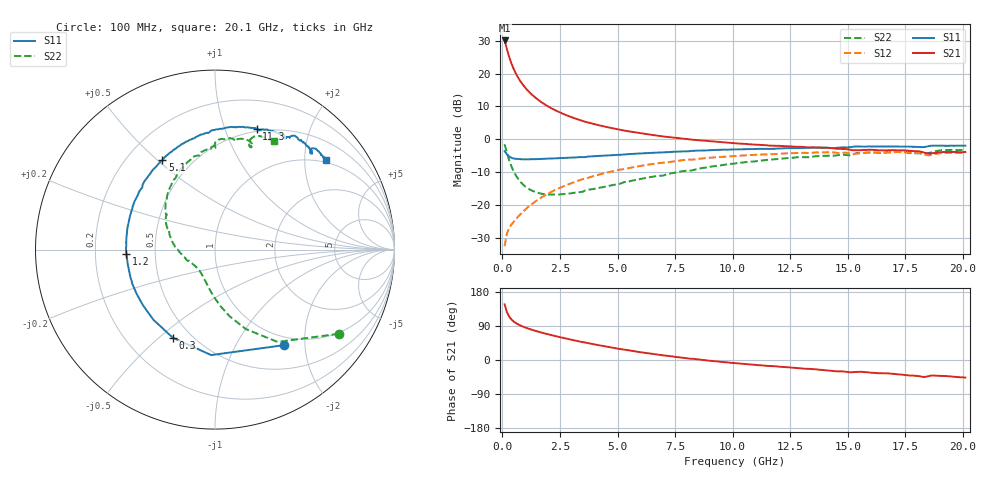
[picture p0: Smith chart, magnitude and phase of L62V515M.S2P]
!  Infineon Technologies AG
! BFR380L3 , PF131585-7, No.6, Th 09.10.01, soldered on pcb-board, measured with PP GSG850
!  Vce=2.5 V,  Ic=15.0 mA
! Common Emitter S-Parameters:  15. November 2001
#  GHz  S  MA  R  50
! f  S11  S21  S12  S22
! GHz  Mag  Ang  Mag  Ang  Mag  Ang  Mag  Ang
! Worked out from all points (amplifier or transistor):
!   201 points, 100 MHz to 20.1 GHz, reference 50 ohm
!   highest |S21| = 30.1 dB at 100 MHz (marker M1)
!   |S21| within 3 dB of that: start of sweep to 214.9 MHz
!   unconditionally stable (mu >= 1): 1.562 GHz to 4.486 GHz
!   at 3.4 GHz: K = 1.02, MAG = 8.2 dB, |S12| = -12.4 dB
!   at 10.1 GHz: K = 0.96, MSG = 1.9 dB, |S12| = -5.1 dB
!   at 20.1 GHz: K = 0.99, MSG = 0.1 dB, |S12| = -4.1 dB
!   S11 on the Smith chart (normalised r, x): 100 MHz: 0.86, -1.60; 300 MHz: 0.40, -0.55; 1.2 GHz: 0.34, -0.02; 5.1 GHz: 0.35, +0.52; 11.3 GHz: 0.47, +1.29; 20.1 GHz: 0.92, +2.52
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0.1  0.656 -54.3  31.89 147.0  0.02344 67.1  0.8341 -34.2
0.2  0.588 -92.1  23.53 126.3  0.03661 55.2  0.6213 -55.9
0.3  0.5441 -115.7  17.81 114.4  0.04449 52.4  0.4746 -68.8
0.4  0.5201 -131.3  14.09 106.8  0.05021 51.8  0.3806 -77.6
0.5  0.5073 -142.2  11.59 101.2  0.05556 52.9  0.3187 -84.2
0.6  0.5016 -150.3  9.81 97.1  0.06122 54.3  0.2758 -89.5
0.7  0.4987 -157.0  8.5 93.6  0.06685 55.5  0.2444 -94.1
0.8  0.4955 -162.0  7.497 90.6  0.07274 56.9  0.2212 -98.1
0.9  0.4929 -166.7  6.699 88.0  0.07869 57.8  0.2033 -101.7
1  0.4929 -170.4  6.063 85.7  0.08481 58.7  0.1897 -105.2
1.2  0.4937 -177.0  5.093 81.4  0.09731 59.9  0.1706 -111.3
1.6  0.4976 172.7  3.87 74.1  0.123 60.9  0.1507 -122.0
2.1  0.5049 162.5  2.996 66.1  0.1556 60.4  0.1435 -133.1
2.7  0.5179 152.2  2.38 57.5  0.1946 58.3  0.1463 -145.1
3.5  0.5327 140.1  1.888 47.0  0.2464 54.3  0.1589 -157.0
5.1  0.5773 120.5  1.392 29.0  0.3434 44.3  0.2089 179.7
6.8  0.6269 103.1  1.122 13.5  0.4318 33.1  0.2764 157.8
10.1  0.6979 78.2  0.866 -8.2  0.5545 11.6  0.4269 126.1
11.3  0.7131 71.0  0.8164 -14.5  0.5849 4.0  0.4752 115.6
13.5  0.7383 60.7  0.7529 -24.1  0.6221 -9.1  0.5429 98.7
16.8  0.7744 48.3  0.6791 -35.5  0.6285 -25.0  0.6314 77.6
20.1  0.7952 39.1  0.6383 -46.3  0.6225 -38.7  0.6876 61.4
